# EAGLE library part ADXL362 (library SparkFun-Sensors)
Analog Devices ADXL362 3-Axis SPI Accelerometer The ADXL362 is an ultralow power, 3-axis MEMS accelerometer that consumes less than 2 μA at a 100 Hz output data rate and 270 nA when in motion triggered wake-up mode. Unlike accelerometers that use power duty cycling to achieve low power consumption, the ADXL362 does not alias input signals by undersampling; it samples the full bandwidth of the sensor at all data rates. Datasheet SparkFun Products SparkFun Triple Axis Accelerometer Breakout - ADXL362 (SEN-11446)
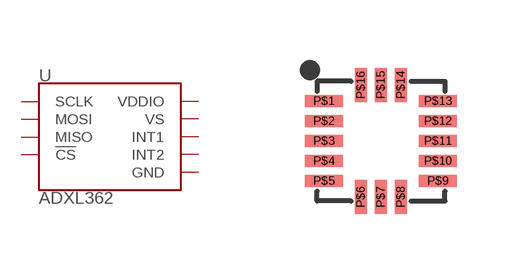
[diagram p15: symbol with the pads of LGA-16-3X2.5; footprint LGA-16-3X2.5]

Designator prefix U

## ADXL362 (PROD_ID: IC-11297)  [LGA-16-3X2.5]
P$1  VDDIO
P$4  SCLK
P$6  MOSI
P$7  MISO
P$8  !CS
P$9  INT2
P$11  INT1
P$12  GND
P$13  GND
P$14  VS
P$16  GND

## Footprint LGA-16-3X2.5 (pad centres in mm)
16-Pin LGA (3 x 3.25 mm) (1:1 footprint) Datasheet Specifications: Pin Count: 16 Dimensions: 3.0 x 3.25 x 1.06 mm Pitch: 0.5 mm Devices Using: ADXL362
smd 0.952 x 0.3: P$1 -1.426,1; P$2 -1.426,0.5; P$3 -1.426,0; P$4 -1.426,-0.5; P$5 -1.426,-1; P$9 1.426,-1; P$10 1.426,-0.5; P$11 1.426,0; P$12 1.426,0.5; P$13 1.426,1
smd 0.3 x 0.851: P$6 -0.5,-1.402; P$7 0,-1.402; P$8 0.5,-1.402; P$14 0.5,1.402; P$15 0,1.402; P$16 -0.5,1.402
